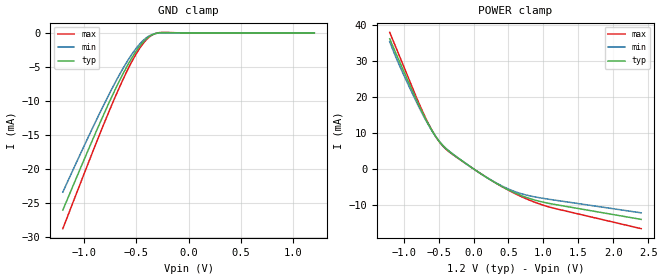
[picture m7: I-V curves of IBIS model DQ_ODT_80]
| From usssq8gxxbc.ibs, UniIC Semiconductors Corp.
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|   Model DQ_ODT_80
[Model] DQ_ODT_80
Model_type Input
Polarity   Non-Inverting
Enable   Active-High
Vinl =  8.300E-01
Vinh =  9.700E-01
C_comp   7.082E-13   7.071E-13   7.120E-13
C_comp_power_clamp   2.986E-13   2.983E-13   3.000E-13
C_comp_gnd_clamp   3.940E-13   3.915E-13   3.982E-13
[Model Spec]
Vinh   9.700E-01   9.250E-01   1.015E+00
Vinl   8.300E-01   7.850E-01   8.750E-01
[Temperature Range]   4.500E+01   9.500E+01   0.000E+00
[Voltage Range]   1.200E+00   1.140E+00   1.260E+00
[C Comp Corner]
C_comp_power_clamp   2.986E-13   3.000E-13   2.983E-13
C_comp_gnd_clamp   3.940E-13   3.915E-13   3.982E-13
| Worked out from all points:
|   GND clamp passes 1 mA (typ) near -0.41 V on its own axis
|   POWER clamp passes 1 mA (typ) near -0.07 V on its own axis
[GND_clamp]
|Voltage   I(typ)   I(min)   I(max)
-1.2V     -26.02mA   -23.38mA   -28.75mA
-875mV    -14.25mA   -12.64mA   -15.92mA
-750mV    -9.946mA   -8.751mA   -11.19mA
-650mV    -6.737mA   -5.871mA   -7.648mA
-575mV    -4.556mA   -3.925mA   -5.213mA
-500mV    -2.665mA   -2.256mA   -3.075mA
-425mV    -1.192mA   -986.7uA   -1.389mA
-375mV    -521.7uA   -429.8uA   -603.8uA
-325mV    -134uA     -120.4uA   -132.5uA
-250mV    37.93uA    19.43uA    76.93uA
1.2V      0A         0A         0A
[POWER_clamp]
|Voltage   I(typ)   I(min)   I(max)
-1.2V     36.21mA    35.38mA    37.99mA
-975mV    26.12mA    25.1mA     27.36mA
-775mV    17.43mA    16.95mA    17.99mA
-650mV    12.56mA    12.37mA    12.76mA
-500mV    7.895mA    7.902mA    7.791mA
-350mV    4.895mA    4.948mA    4.748mA
225mV     -2.851mA   -2.809mA   -2.833mA
450mV     -5.35mA    -5.161mA   -5.409mA
650mV     -7.165mA   -6.703mA   -7.41mA
875mV     -8.674mA   -7.789mA   -9.271mA
1.1V      -9.68mA    -8.518mA   -10.7mA
2.4V      -14.06mA   -12.24mA   -16.64mA
